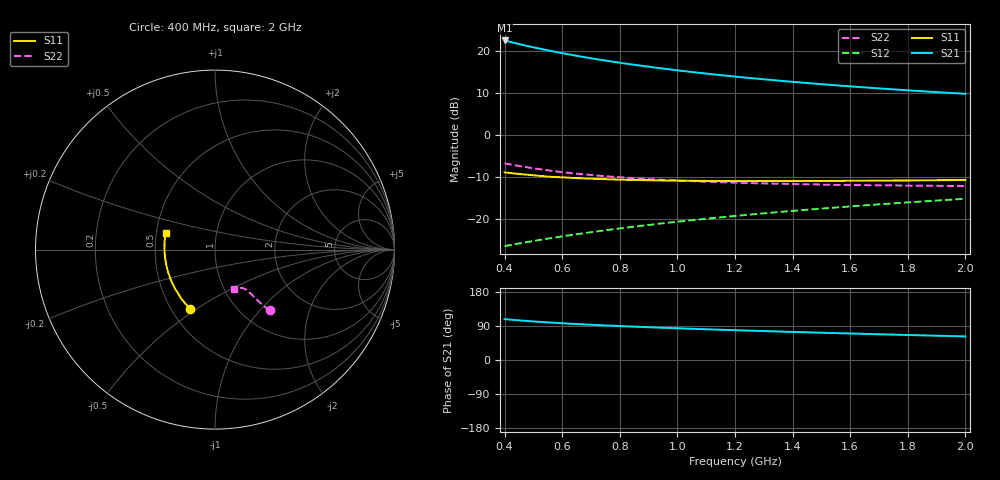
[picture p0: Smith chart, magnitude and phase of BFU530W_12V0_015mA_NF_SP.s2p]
! Filename:  P:\Prog\Test\Noise\ATS_data\Testdata_Net\06 Compressed Noise after Statistics\BFU530W_APM2013_09_A05_12p0V_015mA_NF_CM01_D.sf
! Date/Time: Tue 26/Mar/2013 18:06:01
! BFU530W_APM2013_09_A05_12p0V_1to25mA_NF_CM01_Bias7_R.sf
! Noise Parameter Data File
! BFU530W_APM2013_09_A05_12p0V_1to25mA_NF_CM01
! Date/time: Thu Mar 21 22:54:15 2013
! VAR V_out= 12.000000
! VAR I_out= 14.995000
! VAR V_in= 0.786700
! VAR I_in= 0.136600
! Device data file deembeded for feedlines and parallel
! Original file: \06 Compressed Noise after Statistics\BFU530W_APM2013_09_A05_12p0V_015mA_NF_CM01_R.sf
! Feed-files: PR019V01_070313_Feed1.s2p, PR019V01_070313_Feed2.s2p
! Parallel-file: PR019V01_070313_Par.s2p
# MHz S MA R 50
!  Freq-MHz  S11-mag  S11-arg  S21-mag  S21-arg  S12-mag  S12-arg  S22-mag  S22-arg
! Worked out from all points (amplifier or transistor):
!   37 points, 400 MHz to 2 GHz, reference 50 ohm
!   highest |S21| = 22.5 dB at 400 MHz (marker M1)
!   |S21| within 3 dB of that: start of sweep to 598.2 MHz
!   unconditionally stable (mu >= 1): 1.289 GHz to end of sweep
!   at 500 MHz: K = 0.80, MSG = 23.1 dB, |S12| = -25.3 dB
!   at 1.1 GHz: K = 0.98, MSG = 17.3 dB, |S12| = -20.0 dB
!   at 2 GHz: K = 1.01, MAG = 11.8 dB, |S12| = -15.2 dB
!   lowest NFmin = 0.94 dB at 480 MHz
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400  0.3569 -112.6  13.3 107.9  0.04709 62.3  0.4566 -48.0
420  0.3503 -115.4  12.78 106.5  0.04855 62.5  0.4432 -48.4
433  0.3459 -117.2  12.46 105.7  0.0495 62.6  0.4348 -48.6
460  0.339 -120.6  11.84 104.0  0.05144 62.9  0.4195 -49.0
500  0.3293 -125.6  11.02 101.8  0.05428 63.2  0.3985 -49.5
550  0.3178 -130.7  10.15 99.2  0.05795 63.9  0.3772 -49.8
600  0.3114 -135.6  9.393 97.0  0.06166 64.3  0.3587 -50.1
650  0.3046 -140.0  8.737 94.9  0.06531 64.7  0.3445 -50.4
700  0.2997 -144.1  8.165 93.0  0.06906 65.2  0.3318 -50.6
750  0.296 -147.8  7.662 91.2  0.0728 65.6  0.3205 -50.7
800  0.2918 -151.3  7.217 89.6  0.07662 66.0  0.3121 -51.1
850  0.2899 -154.6  6.824 88.0  0.08042 66.2  0.3032 -51.2
950  0.2853 -160.2  6.151 85.0  0.08819 66.7  0.2905 -51.8
1050  0.2832 -165.4  5.601 82.4  0.09597 67.0  0.2805 -52.3
1150  0.2817 -170.3  5.14 79.9  0.1038 67.2  0.272 -53.0
1200  0.2811 -172.3  4.942 78.7  0.1079 67.2  0.2694 -53.6
1250  0.2811 -174.5  4.754 77.5  0.1118 67.2  0.2658 -54.0
1350  0.2809 -178.2  4.426 75.2  0.12 67.2  0.2615 -55.0
1500  0.282 176.4  4.01 72.0  0.132 66.9  0.2556 -56.9
1650  0.2833 171.4  3.67 69.0  0.1442 66.5  0.2511 -58.8
1750  0.2851 168.6  3.479 67.0  0.1525 66.1  0.2494 -60.1
2000  0.2903 161.5  3.078 62.2  0.1729 65.0  0.2458 -64.2
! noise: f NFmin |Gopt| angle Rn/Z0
400  0.941  0.1281  175.7  0.0899
460  0.9394  0.1376  177.1  0.089
600  0.9645  0.1262  -178.6  0.0947
800  0.9987  0.153  -177.6  0.0881
1000  1.016  0.1678  -174.7  0.0894
1200  1.05  0.1814  -171.9  0.0879
1400  1.091  0.1986  -167.6  0.0852
1600  1.066  0.2179  -165.4  0.0861
1800  1.099  0.2225  -162.9  0.0895
2000  1.159  0.238  -157  0.0906
